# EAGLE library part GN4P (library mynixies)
GN4P tube
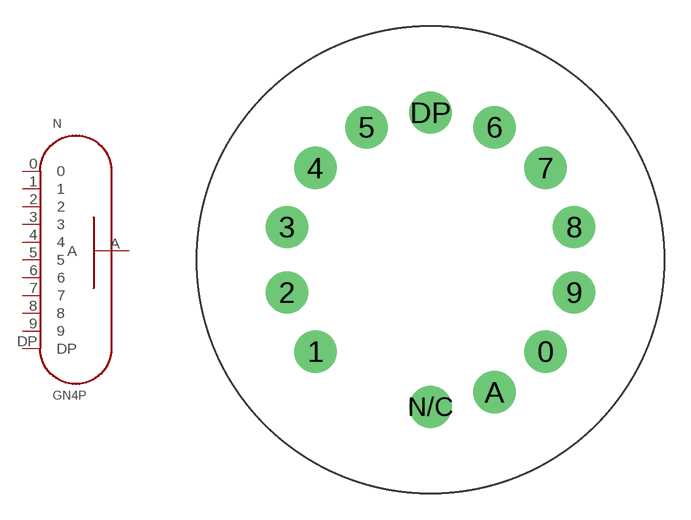
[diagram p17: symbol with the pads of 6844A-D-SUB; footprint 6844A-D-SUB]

Designator prefix N

## GN4P  [6844A-D-SUB]
0  0  pas
1  1  pas
2  2  pas
3  3  pas
4  4  pas
5  5  pas
6  6  pas
7  7  pas
8  8  pas
9  9  pas
A  A  pas
DP  DP  pas

## Footprint 6844A-D-SUB (pad centres in mm)
This footprint uses female D-SUB pins as 'sockets'.
drill 1.6: 0 6.514,-5.194; 1 -6.514,-5.194; 2 -8.122,-1.853; 3 -8.122,1.854; 4 -6.513,5.195; 5 -3.614,7.506; 6 3.615,7.506; 7 6.514,5.194; 8 8.122,1.854; 9 8.122,-1.854; A 3.615,-7.506; DP 0,8.331; N/C 0,-8.331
